[IBIS ver]   4.2
[File name]   tlk6002_noserial.ibs
[File Rev]   1.0
[Date]   Oct 28, 2009
[Source]   TI
[Copyright]   Copyright 2009 Texas Instruments, Inc.
[Notes]   The following is the IBIS model for the TLK6002
   Rev. 1.0:  Initial release
|   Component tlk6002
[Component]   TLK6002
[Manufacturer]  TI
[Package]
| variable   typ   min   max
R_pkg   0.402   0.402   0.402
L_pkg   5.816n   5.816n   5.816n
C_pkg   1.347p   1.347p   1.347p
[Pin]   signal_name   model_name   R_pin   L_pin   C_pin
   A1   DGND   GND
   A2   RDA_12   BSHTLTCSCDVGPBFZ   0.706   9.161n   2.424p
   A3   VDDQA   POWER
   A4   DGND   GND
   A5   REFCLK_0_N   ICLKRX18G   0.629   8.509n   1.767p
   A6   DGND   GND
  A15   DGND   GND
  A16   RDB_7   BSHTLTCSCDVGPBFZ   0.698   9.138n   2.066p
  A17   RDB_13   BSHTLTCSCDVGPBFZ   0.676   9.231n   2.147p
  A18   DGND   GND
   B1   RDA_17   BSHTLTCSCDVGPBFZ   0.674   9.066n   2.519p
   B2   VDDQA   POWER
   B3   RDA_18   BSHTLTCSCDVGPBFZ   0.638   8.952n   2.238p
   B4   DGND   GND
   B5   REFCLK_0_P   ICLKRX18G   0.648   8.988n   1.908p
   B6   DGND   GND
  B15   RDB_6   BSHTLTCSCDVGPBFZ   0.646   9.029n   1.776p
  B16   RDB_12   BSHTLTCSCDVGPBFZ   0.653   9.274n   1.800p
  B17   VDDQB   POWER
  B18   RDB_17   BSHTLTCSCDVGPBFZ   0.674   9.509n   2.204p
   C1   RDA_9   BSHTLTCSCDVGPBFZ   0.638   8.564n   2.089p
   C2   RDA_16   BSHTLTCSCDVGPBFZ   0.632   8.960n   1.964p
   C3   RDA_11   BSHTLTCSCDVGPBFZ   0.612   8.584n   1.891p
   C4   VDDQA   POWER
   C5   DGND   GND
   C6   REFCLK_1_P   ICLKRX18G   0.545   8.002n   1.535p
  C15   VDDQB   POWER
  C16   RDB_11   BSHTLTCSCDVGPBFZ   0.603   8.516n   1.807p
  C17   RDB_16   BSHTLTCSCDVGPBFZ   0.623   8.844n   1.925p
  C18   RDB_9   BSHTLTCSCDVGPBFZ   0.631   9.129n   2.169p
   D1   RDA_19   BSHTLTCSCDVGPBFZ   0.588   7.871n   2.143p
   D2   DGND   GND
   D3   RDA_10   BSHTLTCSCDVGPBFZ   0.556   7.668n   1.733p
   D4   RDA_7   BSHTLTCSCDVGPBFZ   0.549   7.686n   1.728p
   D5   DGND   GND
   D6   REFCLK_1_N   ICLKRX18G   0.565   7.892n   1.778p
  D14   CS_N   BC1825ETHYFZ   0.567   8.657n   1.675p
  D15   RDB_5   BSHTLTCSCDVGPBFZ   0.537   7.817n   1.640p
  D16   RDB_10   BSHTLTCSCDVGPBFZ   0.555   7.935n   1.535p
  D17   DGND   GND
  D18   RDB_19   BSHTLTCSCDVGPBFZ   0.593   7.947n   1.998p
   E1   VDDQA   POWER
   E2   RDA_15   BSHTLTCSCDVGPBFZ   0.534   7.746n   1.751p
   E3   DGND   GND
   E4   RDA_6   BSHTLTCSCDVGPBFZ   0.505   7.578n   1.662p
   E5   RDA_2   BSHTLTCSCDVGPBFZ   0.502   7.521n   1.517p
  E14   SDI   BC1825ETHYFZ   0.502   7.913n   1.531p
  E15   RDB_4   BSHTLTCSCDVGPBFZ   0.511   7.518n   1.535p
  E16   DGND   GND
  E17   RDB_18   BSHTLTCSCDVGPBFZ   0.536   7.840n   1.377p
  E18   VDDQB   POWER
   F1   RXCLK_A   BSHTLTCSCDVGPBFZ   0.518   6.722n   1.594p
   F2   RDA_14   BSHTLTCSCDVGPBFZ   0.499   7.023n   1.649p
   F3   RDA_13   BSHTLTCSCDVGPBFZ   0.504   7.194n   1.603p
   F4   RDA_8   BSHTLTCSCDVGPBFZ   0.462   6.846n   1.484p
   F5   VDDQA   POWER
  F14   VDDQB   POWER
  F15   RDB_8   BSHTLTCSCDVGPBFZ   0.463   6.840n   1.276p
  F16   RDB_15   BSHTLTCSCDVGPBFZ   0.512   7.528n   1.487p
  F17   RDB_14   BSHTLTCSCDVGPBFZ   0.493   7.231n   1.512p
  F18   RXCLK_B   BSHTLTCSCDVGPBFZ   0.528   6.752n   1.789p
   G1   DGND   GND
   G2   VDDQA   POWER
   G3   RDA_4   BSHTLTCSCDVGPBFZ   0.452   6.693n   1.546p
   G4   RDA_5   BSHTLTCSCDVGPBFZ   0.414   6.260n   1.410p
   G5   RDA_0   BSHTLTCSCDVGPBFZ   0.398   6.046n   1.293p
  G14   RDB_0   BSHTLTCSCDVGPBFZ   0.399   5.897n   1.140p
  G15   RDB_1   BSHTLTCSCDVGPBFZ   0.441   6.652n   1.516p
  G16   RDB_3   BSHTLTCSCDVGPBFZ   0.442   6.587n   1.317p
  G17   VDDQB   POWER
  G18   DGND   GND
   H1   TDA_19   BSHTLTCSCDVGPBFZ   0.469   6.544n   1.358p
   H2   TDA_17   BSHTLTCSCDVGPBFZ   0.421   6.338n   1.308p
   H3   DGND   GND
   H4   RDA_3   BSHTLTCSCDVGPBFZ   0.414   6.274n   1.316p
   H5   RDA_1   BSHTLTCSCDVGPBFZ   0.355   5.181n   1.150p
  H13   SCL   BC1825ETHYFZ   0.397   5.987n   1.172p
  H14   DGND   GND
  H15   RDB_2   BSHTLTCSCDVGPBFZ   0.429   6.128n   1.351p
  H16   DGND   GND
  H17   TDB_18   BSHTLTCSCDVGPBFZ   0.405   6.269n   1.488p
  H18   TDB_16   BSHTLTCSCDVGPBFZ   0.467   6.553n   1.421p
   J1   TDA_14   BSHTLTCSCDVGPBFZ   0.439   5.978n   1.344p
   J2   TDA_15   BSHTLTCSCDVGPBFZ   0.406   5.949n   1.141p
   J3   TDA_18   BSHTLTCSCDVGPBFZ   0.420   5.903n   1.019p
   J4   VDDQA   POWER
   J5   DGND   GND
   J6   CLK_OUT_P   OCML11G   0.335   5.081n   1.108p
   J7   CLK_OUT_N   OCML11G   0.307   4.847n   1.183p
  J14   RESRB   NC   0.372   4.670n   1.099p
  J15   VDDQB   POWER
  J16   TDB_17   BSHTLTCSCDVGPBFZ   0.399   5.643n   1.149p
  J17   TDB_19   BSHTLTCSCDVGPBFZ   0.403   5.919n   1.244p
  J18   TDB_5   BSHTLTCSCDVGPBFZ   0.431   6.058n   1.240p
   K1   VDDQA   POWER
   K2   DGND   GND
   K3   TDA_8   BSHTLTCSCDVGPBFZ   0.421   5.966n   1.155p
   K4   TDA_16   BSHTLTCSCDVGPBFZ   0.380   5.304n   0.985p
   K5   TDA_13   BSHTLTCSCDVGPBFZ   0.362   5.037n   1.084p
   K6   DGND   GND
   K8   RESRA   NC   0.259   3.448n   0.740p
   K9   VPP   POWER   0.120   2.935n   0.836p
  K10   GPI1   IC18THY   0.246   3.737n   0.846p
  K11   PRTAD1   BC1850BTHYFZ   0.252   3.417n   0.723p
  K12   PRTAD2   BC1850BTHYFZ   0.291   4.036n   0.801p
  K13   SDO   BC1825ETHYFZ   0.386   5.884n   1.223p
  K14   DGND   GND
  K15   TDB_15   BSHTLTCSCDVGPBFZ   0.345   4.605n   0.977p
  K16   TDB_14   BSHTLTCSCDVGPBFZ   0.430   5.966n   1.205p
  K17   DGND   GND
  K18   VDDQB   POWER
   L1   VREFTA   POWER   0.408   5.556n   1.229p
   L2   DGND   GND
   L3   TDA_12   BSHTLTCSCDVGPBFZ   0.394   5.320n   1.109p
   L4   VDDQA   POWER
   L5   TDA_11   BSHTLTCSCDVGPBFZ   0.261   3.559n   0.862p
   L6   DVDD   POWER
   L7   VDDQA   POWER
   L8   VDDQA   POWER
   L9   DVDD   POWER
  L10   VDDO1   POWER   0.101   1.963n   1.006p
  L11   PRTAD0   BC1850BTHYFZ   0.259   3.316n   0.770p
  L12   VDDQB   POWER
  L13   DVDD   POWER
  L14   TDB_13   BSHTLTCSCDVGPBFZ   0.290   3.985n   0.857p
  L15   VDDQB   POWER
  L16   TDB_12   BSHTLTCSCDVGPBFZ   0.387   5.583n   1.088p
  L17   VDDQB   POWER
  L18   VREFTB   POWER   0.388   5.574n   1.052p
   M1   RESTA   NC   0.399   5.554n   1.167p
   M2   TDA_5   BSHTLTCSCDVGPBFZ   0.395   5.471n   1.196p
   M3   TDA_10   BSHTLTCSCDVGPBFZ   0.377   5.163n   1.100p
   M4   TDA_9   BSHTLTCSCDVGPBFZ   0.243   3.523n   0.708p
   M5   TDA_7   BSHTLTCSCDVGPBFZ   0.377   5.106n   1.078p
   M6   VDDQA   POWER
   M7   DGND   GND
   M8   PRTAD3   BC1850BTHYFZ   0.380   4.840n   0.984p
   M9   DGND   GND
  M10   DVDD   POWER
  M11   DGND   GND
  M12   DVDD   POWER
  M13   VDDQB   POWER
  M14   TDB_11   BSHTLTCSCDVGPBFZ   0.322   4.594n   0.905p
  M15   TDB_9   BSHTLTCSCDVGPBFZ   0.381   5.547n   1.042p
  M16   TDB_10   BSHTLTCSCDVGPBFZ   0.360   5.187n   1.078p
  M17   TDB_4   BSHTLTCSCDVGPBFZ   0.397   5.506n   1.323p
  M18   RESTB   NC   0.363   5.101n   1.006p
   N1   VDDQA   POWER
   N2   DGND   GND
   N3   TDA_6   BSHTLTCSCDVGPBFZ   0.395   5.000n   1.118p
   N4   DGND   GND
   N5   TDA_2   BSHTLTCSCDVGPBFZ   0.279   3.786n   0.874p
   N6   DVDD   POWER
   N7   DGND   GND
   N8   DGND   GND
  N10   DGND   GND
  N11   DGND   GND
  N12   DGND   GND
  N13   DVDD   POWER
  N14   TDB_7   BSHTLTCSCDVGPBFZ   0.274   4.034n   0.895p
  N15   DGND   GND
  N16   TDB_6   BSHTLTCSCDVGPBFZ   0.401   5.022n   1.187p
  N17   DGND   GND
  N18   VDDQB   POWER
   P1   TXCLK_A   BSHTLTCSCDVGPBFZ   0.393   4.894n   1.309p
   P2   TDA_4   BSHTLTCSCDVGPBFZ   0.410   5.414n   1.327p
   P3   VDDQA   POWER
   P4   TDA_3   BSHTLTCSCDVGPBFZ   0.302   4.031n   0.838p
   P5   TDA_0   BSHTLTCSCDVGPBFZ   0.399   5.425n   1.266p
   P6   VDDQA   POWER
   P7   DGND   GND
   P8   DGND   GND
   P9   DGND   GND
  P10   DGND   GND
  P11   DGND   GND
  P12   DGND   GND
  P13   VDDQB   POWER
  P14   TDB_1   BSHTLTCSCDVGPBFZ   0.361   4.936n   1.066p
  P15   TDB_2   BSHTLTCSCDVGPBFZ   0.349   5.190n   1.226p
  P16   VDDQB   POWER
  P17   TDB_8   BSHTLTCSCDVGPBFZ   0.401   5.324n   1.060p
  P18   TDB_0   BSHTLTCSCDVGPBFZ   0.405   5.563n   1.186p
   R1   DGND   GND
   R2   TDA_1   BSHTLTCSCDVGPBFZ   0.380   5.000n   1.282p
   R3   TMS   IC18THYPUFZ   0.353   5.334n   1.089p
   R4   GPI0   IC18THY   0.254   4.115n   0.893p
   R5   DGND   GND
   R6   REFCLK_A_SEL   IC18THY   0.290   4.359n   0.882p
   R7   VDDO3   POWER   0.057   1.568n   1.042p
   R8   DVDD   POWER
   R9   AGND   GND
  R10   DVDD   POWER
  R11   AGND   GND
  R12   DVDD   POWER
  R13   VDDO2   POWER   0.052   1.530n   1.061p
  R14   TDO   OC1850BTFZ   0.251   4.117n   1.050p
  R15   TDI   IC18THYPUFZ   0.278   4.301n   1.063p
  R16   PRBS_EN   IC18THY   0.338   5.496n   1.241p
  R17   TDB_3   BSHTLTCSCDVGPBFZ   0.395   5.277n   1.173p
  R18   DGND   GND
   T1   MDC   IC18THY   0.376   5.248n   1.409p
   T2   REFCLK_B_SEL   IC18THY   0.371   5.628n   1.319p
   T3   TRST_N   IC18THYPDFZ   0.341   5.224n   1.232p
   T4   RATE_A1   IC18THY   0.306   4.922n   1.084p
   T5   DVDD   POWER
   T6   PD_TRXA_N   IC18THY   0.253   4.215n   0.827p
   T7   VDDRA   POWER   0.209   3.215n   0.740p
   T8   VDDD   POWER   0.096   1.478n   1.541p
   T9   AVDD   POWER
  T10   AVDD   POWER
  T11   VDDD   POWER   0.096   1.478n   1.541p
  T12   VDDRB   POWER   0.207   2.974n   0.813p
  T13   AVDD   POWER
  T14   AGND   GND
  T15   CLK_OUT_SEL   IC18THY   0.324   5.018n   1.250p
  T16   TCK   IC18THY   0.339   5.271n   1.242p
  T17   TESTEN   IC18THY   0.373   5.365n   1.323p
  T18   TXCLK_B   BSHTLTCSCDVGPBFZ   0.399   4.877n   1.280p
   U1   DGND   GND
   U2   MDIO   BC1825ETHYFZ   0.400   5.758n   1.390p
   U3   RATE_A0   IC18THY   0.390   6.111n   1.319p
   U4   LOSA   OC1840DTFZ   0.360   6.090n   1.329p
|  U5   AMUXA   Not modeled
   U6   AVDD   POWER
   U7   AGND   GND
|  U8   RXAN   Not modeled
|  U9   RXAP   Not modeled
  U10   AGND   GND
  U11   AVDD   POWER
| U12   TXBP   Not modeled
| U13   TXBN   Not modeled
  U14   AVDD   POWER
  U15   PD_TRXB_N   IC18THY   0.384   6.835n   1.566p
  U16   RATE_B2   IC18THY   0.342   5.930n   1.226p
  U17   RATE_B1   IC18THY   0.394   6.581n   1.691p
  U18   RATE_B0   IC18THY   0.448   7.227n   2.005p
   V1   RESET_N   IC18THY   0.424   6.306n   1.601p
   V2   RATE_A2   IC18THY   0.404   6.174n   1.490p
   V3   PRBSA_PASS   OC1840DTFZ   0.356   5.921n   1.322p
   V4   CODEA_EN   IC18THY   0.349   6.056n   1.383p
   V5   AGND   GND
|  V6   TXAN   Not modeled
|  V7   TXAP   Not modeled
   V8   VDDT   POWER   0.059   1.169n   3.346p
   V9   AGND   GND
| V10   RXBP   Not modeled
| V11   RXBN   Not modeled
  V12   VDDT   POWER   0.059   1.169n   3.346p
  V13   AGND   GND
| V14   AMUXB   Not modeled
  V15   PRTAD4   BC1850BTHYFZ   0.371   6.179n   1.541p
  V16   CODEB_EN   IC18THY   0.395   6.572n   1.495p
  V17   LOSB   OC1840DTFZ   0.431   6.912n   1.813p
  V18   PRBSB_PASS   OC1840DTFZ   0.425   7.223n   1.884p
[Model Selector] BSHTLTCSCDVGPBFZ
NOSR0_10PER_1P8  Fast slew rate, 10% supply tolerance, 1.8 nominal supply
SR0_10PER_1P8  Slow slew rate, 10% supply tolerance, 1.8 nominal supply
NOSR0_5PER_1P5  Fast slew rate, 5% supply tolerance, 1.5 nominal supply
SR0_5PER_1P5  Slow slew rate, 5% supply tolerance, 1.5 nominal supply
NOSR0_10PER_1P5  Fast slew rate, 10% supply tolerance, 1.5 nominal supply
SR0_10PER_1P5  Slow slew rate, 10% supply tolerance, 1.5 nominal supply
NOSR0_5PER_1P8  Fast slew rate, 5% supply tolerance, 1.8 nominal supply
SR0_5PER_1P8  Slow slew rate, 5% supply tolerance, 1.8 nominal supply
10P_HALFT_1P8  half termination strength, 10% supply tolerance, 1.8 nominal supply
10P_NOT_1P8  no termination, 10% supply tolerance, 1.8 nominal supply
10P_FULLT_1P8  full termination strength, 10% supply tolerance, 1.8 nominal supply
5P_HALFT_1P5  half termination strength, 5% supply tolerance, 1.5 nominal supply
5P_NOT_1P5  no termination, 5% supply tolerance, 1.5 nominal supply
5P_FULLT_1P5  full termination strength, 5% supply tolerance, 1.5 nominal supply
10P_HALFT_1P5  half termination strength, 10% supply tolerance, 1.5 nominal supply
10P_NOT_1P5  no termination, 10% supply tolerance, 1.5 nominal supply
10P_FULLT_1P5  full termination strength, 10% supply tolerance, 1.5 nominal supply
5P_HALFT_1P8  half termination strength, 5% supply tolerance, 1.8 nominal supply
5P_NOT_1P8  no termination, 5% supply tolerance, 1.8 nominal supply
5P_FULLT_1P8  full termination strength, 5% supply tolerance, 1.8 nominal supply
| Models and submodels in the file (29): BC1825ETHYFZ (I/O), BC1850BTHYFZ (I/O), NOSR0_10PER_1P8 (3-state), SR0_10PER_1P8 (3-state), NOSR0_5PER_1P5 (3-state), SR0_5PER_1P5 (3-state), NOSR0_10PER_1P5 (3-state), SR0_10PER_1P5 (3-state), NOSR0_5PER_1P8 (3-state), SR0_5PER_1P8 (3-state), 10P_HALFT_1P8 (Input), 10P_NOT_1P8 (Input), 10P_FULLT_1P8 (Input), 5P_HALFT_1P5 (Input), 5P_NOT_1P5 (Input), 5P_FULLT_1P5 (Input), 10P_HALFT_1P5 (Input), 10P_NOT_1P5 (Input), 10P_FULLT_1P5 (Input), 5P_HALFT_1P8 (Input), 5P_NOT_1P8 (Input), 5P_FULLT_1P8 (Input), IC18THY (Input), IC18THYPDFZ (Input), IC18THYPUFZ (Input), ICLKRX18G (Input), OC1840DTFZ (3-state), OC1850BTFZ (3-state), OCML11G (Output)
